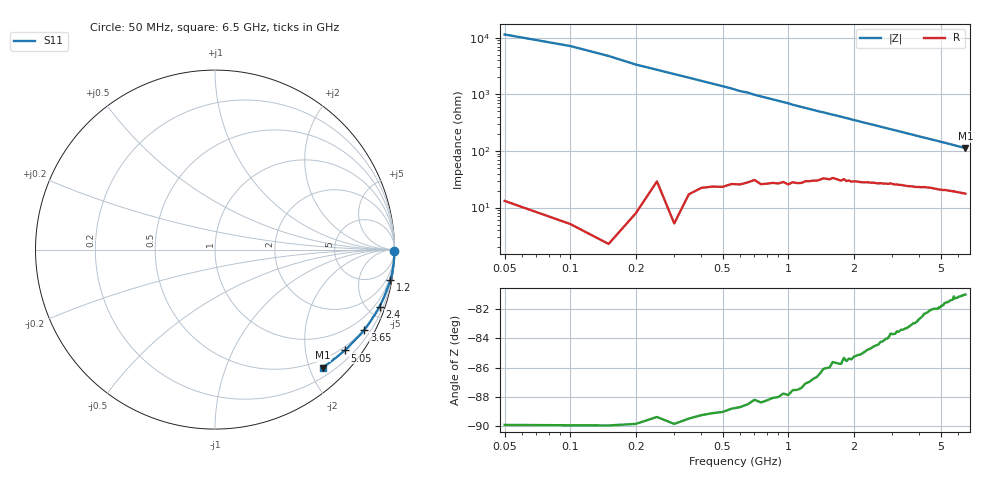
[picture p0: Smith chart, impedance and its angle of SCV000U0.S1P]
! Infineon Technologies  Discrete & RF Semiconductors
! BAR63-02L
! Si PIN Diode in TSLP-2
! VR = 0 V
! S-Parameters:  March  2002
# GHz  S  MA  R  50
!  f  S11
! GHz  MAG  ANG
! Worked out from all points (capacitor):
!   130 points, 50 MHz to 6.5 GHz, reference 50 ohm
!   read as one part to ground: C = 222 fF near 50 MHz
!   lowest |Z| = 112 ohm at 6.5 GHz (marker M1)
!   S11 on the Smith chart (normalised r, x): 50 MHz: open; 1.2 GHz: 1, -12; 2.4 GHz: 0.55, -5.89; 3.65 GHz: 0.48, -3.93; 5.05 GHz: 0.41, -2.86; 6.5 GHz: 0.35, -2.22
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0.05  1 -0.5
0.1  1 -0.8
0.2  0.9999 -1.7
0.5  0.9988 -4.1
0.6  0.998 -5.0
0.65  0.9976 -5.3
0.7  0.9969 -5.8
0.9  0.9956 -7.4
1.2  0.9913 -9.9
1.4  0.9875 -11.5
1.7  0.9824 -13.7
1.85  0.9802 -14.9
1.9  0.979 -15.2
2  0.9772 -16.1
2.4  0.97 -19.1
2.5  0.968 -19.8
2.9  0.9593 -22.8
3.3  0.9513 -25.6
3.65  0.9444 -28.2
3.85  0.9402 -29.7
4.1  0.9339 -31.4
4.9  0.9181 -36.8
5.05  0.9149 -37.9
5.7  0.9028 -42.2
5.75  0.8998 -42.6
5.85  0.9002 -43.2
6  0.8976 -44.3
6.5  0.8897 -47.6
